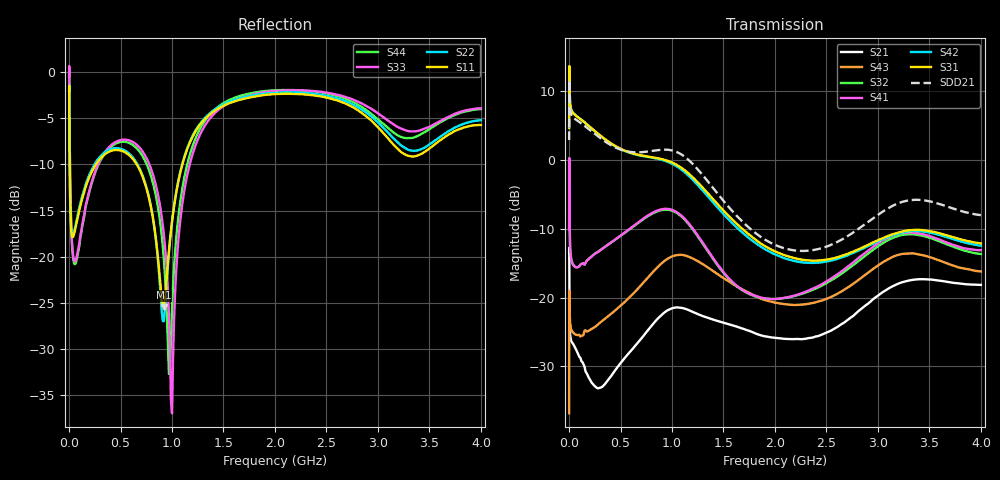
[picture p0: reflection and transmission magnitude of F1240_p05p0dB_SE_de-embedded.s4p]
! Integrated Device Technology
! Corporate Headquarters
! 6024 Silver Creek Valley Road
! San Jose, CA 95138  USA
! Phone:  1-408-284-8200
! Toll Free:  1-800-223-1366
! Webpage:  http://www.idt.com/
! Timing and RF Division
! 515 Groton Road, Suite 102
! Westford, MA 01886-6024
! Device:  F1240
! Description: Dual Intermediate Frequency Digital Variable Gain Amplifier
! Frequency:  10.0 -  500.00 MHz
! Package:  5x5 mm QFN Plastic Package: 32 pin
! Ports:  8 RF, 20 DC
!  Pin  1  = GA3 / Data  Pin 17  = RF OUT_B+
!  Pin  2  = GA4 / CLK  Pin 18  = RF OUT_B-
!  Pin  3  = GA5  Pin 19  = STBY_B
!  Pin  4  = VMODE  Pin 20  = Ground
!  Pin  5  = No Connect  Pin 21  = Ground
!  Pin  6  = GB5  Pin 22  = STB_A
!  Pin  7  = GB4  Pin 23  = RF OUT_A-  = Port 4
!  Pin  8  = GB3  Pin 24  = RF OUT_A+  = Port 3
!  Pin  9  = GB2  Pin 25  = GA0
!  Pin 10  = GB1  Pin 26  = ISET_A
!  Pin 11  = RF IN_B+  Pin 27  = VCC
!  Pin 12  = RF IN_B-  Pin 28  = Ground
!  Pin 13  = Ground  Pin 29  = RF IN_A-  = Port 2
!  Pin 14  = VCC  Pin 30  = RF IN_A+  = Port 1
!  Pin 15  = ISET_B  Pin 31  = GA1
!  Pin 16  = GB0  Pin 32  = GA2 / CSb
! Gain  = +19.5 dB
! State  = 1
! Voltage  = +5.00 V
! Current  = 85.292 mA (one channel only)
! Temperture  =  +25 C
! Test Date  =  2017-10-18
! Board  =  EB4031
! Data:  The device was measured on a custom evaluation board which has
!  individual transmission lines to the RF pins.  Data was collected
!  using a calibrated network analyzer.  The evaluation board was
!  de-embedded using Automatic Fixture Removal.
!  The reference plane is the edge of the package pin.
!  Only Channel A was measured.
!  This data is in single-ended operation.  If your needs are balanced
!  or differential S-parameters then this file needs to be used a
!  linear simulator.
! File Date:  2017-11-10  MJV
! Note:
!  Integrated Device Technology supplies this data as a sample of measured
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# Hz S dB R 100
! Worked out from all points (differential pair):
!   410 points, 500 kHz to 4 GHz, reference 100 ohm
!   strongest paths, dB at 500 kHz, 930 MHz, 1.96 GHz, 2.98 GHz, 4 GHz:
!     S31: 4.7, 0.0, -13.0, -11.8, -12.1
!     S42: 4.6, -0.1, -13.4, -12.0, -12.5
!     S41: -10.1, -7.1, -20.2, -12.4, -13.1
!     S32: -10.1, -7.2, -20.2, -12.8, -13.7
!     S43: -36.8, -14.6, -20.6, -15.6, -16.2
!     S21: -13.4, -22.1, -25.8, -19.9, -18.2
!   taken as a pair (ports 1,2 in; 3,4 out), SDD21 dB: 2.9, 1.5, -12.1, -8.2, -8.0
!   lowest |S11| = -25.5 dB at 920 MHz (marker M1), VSWR 1.11, Z = 91.5 - j5.62 ohm
!   |S11| at or under -10 dB: 6.53 MHz to 260.3 MHz (253.8 MHz wide, 190 % of centre); 656.7 MHz to 1.101 GHz (444.2 MHz wide, 50.5 % of centre)
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500000  -2.04 -5.5  -13.42 -5.8  -28.07 82.5  -44.99 79.3
        -13.43 -5.8  -2.04 -5.5  -45.00 77.9  -28.08 83.7
        4.65 -105.4  -10.12 -104.0  -0.46 1.3  -36.87 -67.3
        -10.10 -102.8  4.64 -104.3  -36.83 -67.1  -0.47 3.6
2500000  -3.37 -50.5  -16.35 -58.1  -16.77 32.5  -35.68 -3.0
         -16.37 -58.1  -3.35 -50.5  -35.63 -3.3  -16.78 32.7
         13.26 -175.8  -1.32 162.9  -0.82 -50.0  -19.03 -148.7
         -1.36 162.9  13.24 -175.5  -19.01 -148.8  -0.88 -49.7
4500000  -7.62 -67.3  -22.09 -52.8  -16.43 14.7  -39.10 -21.4
         -22.10 -52.7  -7.57 -67.4  -39.05 -21.7  -16.44 14.8
         10.83 166.0  -7.74 140.0  -4.89 -74.1  -21.23 179.9
         -7.80 140.0  10.82 166.2  -21.18 179.8  -4.95 -74.1
3e7  -17.88 -88.2  -26.54 -20.8  -16.89 -8.2  -43.26 6.1
     -26.55 -21.0  -17.70 -88.9  -43.31 6.3  -16.87 -8.1
     7.00 161.6  -14.93 140.5  -18.83 -122.3  -24.97 160.7
     -14.96 141.0  7.03 161.7  -24.89 160.8  -19.04 -122.8
1.9e8  -11.57 -129.4  -31.53 -42.9  -18.42 -48.9  -36.13 10.6
       -31.61 -42.3  -11.31 -130.4  -36.16 11.4  -18.43 -49.1
       4.96 111.4  -14.37 52.3  -13.14 -119.0  -24.98 101.1
       -14.42 52.6  4.95 110.8  -24.84 100.9  -13.26 -118.2
9.2e8  -25.48 -144.8  -22.43 -103.0  -18.26 161.2  -27.84 -146.5
       -22.25 -106.7  -27.02 -142.8  -27.95 -140.0  -18.60 160.0
       0.05 -75.0  -7.24 -179.3  -17.54 136.1  -15.17 -85.9
       -7.12 177.5  -0.06 -77.1  -14.76 -86.8  -20.21 141.3
4e9  -5.73 -142.0  -18.18 98.4  -23.02 -62.3  -23.98 -43.7
     -18.15 98.0  -5.20 -140.8  -24.75 -26.5  -24.62 -56.6
     -12.12 25.2  -13.67 -86.1  -3.92 -137.4  -17.33 72.6
     -13.11 -100.1  -12.46 31.3  -16.20 58.7  -4.00 -146.3
